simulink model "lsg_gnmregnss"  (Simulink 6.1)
settings: Solver=ode45  StartTime=0.0  StopTime=Tstop  MaxStep=step_max  RelTol=1e-3
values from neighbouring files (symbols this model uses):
  A = [ -RA/LA           -CE*PsiN/LA  ;         CM*PsiN/(2*pi*J) 0           ;      ]    [lsg_gnmregnss_ini.m]
  B = [  1/LA    0          ;         0      -1/(2*pi*J) ;      ]    [lsg_gnmregnss_ini.m]
  C = [  1  0 ;         0  1        ]    [lsg_gnmregnss_ini.m]
  CE = 2*pi*CM    (= 240.017678734)    [gnm_i.m]
  CM = 38.2    [gnm_i.m]
  D = zeros(size(C*B))    [lsg_gnmregnss_ini.m]
  int_regi = 0    [gnmregi_i.m]
  int_regn = 0    [lsg_gnmregnss_ini.m]    (also in gnmregn_i.m)
  J = 0.012    [gnm_i.m]
  MW = 0    [gnm_i.m]    (also in lsg_gnmregnss_ini.m = 100; gnmbeobreg_i.m = 10; gnmbeob_i.m = 10; gnmregn_i.m = 100)
  N_soll = 500/60    (= 8.33333333333)    [lsg_gnmregnss_ini.m]    (also in gnmbeobreg_i.m; gnmregn_i.m)
  PsiN = 0.04    [gnm_i.m]
  RA = 0.250    (= 0.25)    [gnm_i.m]
  T_MW = 0    [gnm_i.m]    (also in lsg_gnmregnss_ini.m = 0.1; gnmbeobreg_i.m = 0.4; gnmbeob_i.m = 0.4; gnmregn_i.m = 0.1)
  T_Nsoll = 0.40    (= 0.4)    [lsg_gnmregnss_ini.m]    (also in gnmbeobreg_i.m = 0.8; gnmregn_i.m)
  T_Ri = TA    [gnmregi_i.m]
  T_Rn = 4^2*2*T_t    [lsg_gnmregnss_ini.m]    (also in gnmregn_i.m = 4*2*T_t)
  T_t = 0.0001    [gnmregi_i.m]    (also in gnmbeobreg_i.m; gnmbeob_i.m)
  TA = LA / RA    (= 0.016)    [gnm_i.m]
  V_Ri = LA / (2*T_t)    [gnmregi_i.m]
  V_Rn = 2*pi*J / (CM*PsiN*4*2*T_t)    [lsg_gnmregnss_ini.m]    (also in gnmregn_i.m = 2*pi*J / (CM*PsiN*2*2*T_t))

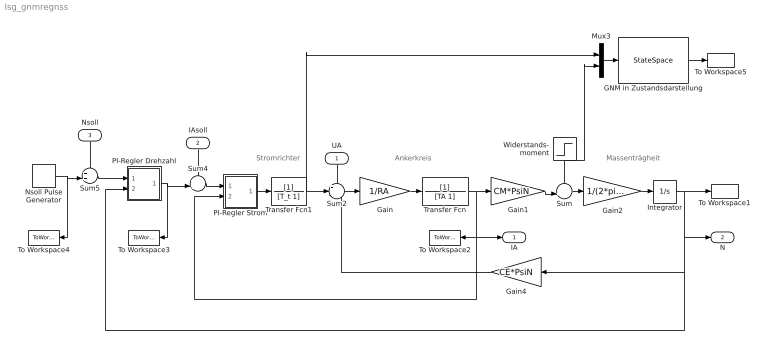
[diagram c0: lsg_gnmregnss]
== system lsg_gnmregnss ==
  note: Massenträgheit
  note: Ankerkreis
  note: Stromrichter
  UA : Inport  Orientation=down  Port=1  LatchInput=off
  IAsoll : Inport  Orientation=down  Port=2  PortDimensions=1  LatchInput=off
  Nsoll : Inport  Orientation=down  Port=3  PortDimensions=1  LatchInput=off
  GNM in Zustandsdarstellung : StateSpace  A=A  B=B  C=C  D=D
  Gain : Gain  Gain=1/RA
  Gain1 : Gain  Gain=CM*PsiN
  Gain2 : Gain  Gain=1/(2*pi*J)
  Gain4 : Gain  Orientation=left  Gain=CE*PsiN
  Integrator : Integrator
  Mux3 : Mux  Inputs=2
  Nsoll Pulse Generator : DiscretePulseGenerator  PulseType=Time based  Amplitude=N_soll  Period=T_Nsoll  PulseWidth=50
  PI-Regler Drehzahl : Subsystem  mask(PI-Regler){V_R=V_Rn, T_n=T_Rn, int_R=int_regn}
      mask prompts: V_R "Verstärkungsfaktor V_R"; T_n "Nachstellzeit T_n"; int_R "Startwert Regler-Integrator"
      mask help: 1 + s*T_n 1 + s*T_n Übertragungsfunktion: G_R = V_R * ------------------ = K_R * ------------------ s*T_n s
  PI-Regler Strom : Subsystem  mask(PI-Regler){V_R=V_Ri, T_n=T_Ri, int_R=int_regi}
      mask prompts: V_R "Verstärkungsfaktor V_R"; T_n "Nachstellzeit T_n"; int_R "Startwert Regler-Integrator"
      mask help: 1 + s*T_n 1 + s*T_n Übertragungsfunktion: G_R = V_R * ------------------ = K_R * ------------------ s*T_n s
  Sum : Sum  Inputs=-+|
  Sum2 : Sum  Inputs=++-
  Sum4 : Sum  Inputs=++|
  Sum5 : Sum  Inputs=++|
  To Workspace1 : ToWorkspace  VariableName=N  SampleTime=-1  SaveFormat=Array
  To Workspace2 : ToWorkspace  VariableName=IA  SampleTime=-1  SaveFormat=Array
  To Workspace3 : ToWorkspace  VariableName=IAsoll  SampleTime=-1  SaveFormat=Array
  To Workspace4 : ToWorkspace  VariableName=Nsoll  SampleTime=-1  SaveFormat=Array
  To Workspace5 : ToWorkspace  VariableName=yss  SampleTime=-1  SaveFormat=Array
  Transfer Fcn : TransferFcn  Denominator=[TA 1]
  Transfer Fcn1 : TransferFcn  Denominator=[T_t 1]
  Widerstands- moment : Step  Orientation=down  Time=T_MW  After=MW  SampleTime=0
  IA : Outport
  N : Outport  Port=2
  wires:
  PI-Regler Strom/1(Reglerausgang) -> Transfer Fcn1/1
  Gain/1 -> Transfer Fcn/1
  Sum2/1 -> Gain/1
  Gain1/1 -> Sum/2
  Widerstands- moment/1 -> Sum/1, Mux3/2
  Sum/1 -> Gain2/1
  Gain2/1 -> Integrator/1
  Integrator/1 -> To Workspace1/1, N/1, Gain4/1, PI-Regler Drehzahl/2(Istwert)
  UA/1 -> Sum2/1
  Gain4/1 -> Sum2/3
  Transfer Fcn/1 -> To Workspace2/1, IA/1, PI-Regler Strom/2(Istwert), Gain1/1
  Transfer Fcn1/1 -> Sum2/2, Mux3/1
  IAsoll/1 -> Sum4/1
  Sum4/1 -> PI-Regler Strom/1(Sollwert)
  PI-Regler Drehzahl/1(Reglerausgang) -> Sum4/2, To Workspace3/1
  Nsoll/1 -> Sum5/1
  Sum5/1 -> PI-Regler Drehzahl/1(Sollwert)
  Nsoll Pulse Generator/1 -> To Workspace4/1, Sum5/2
  GNM in Zustandsdarstellung/1 -> To Workspace5/1
  Mux3/1 -> GNM in Zustandsdarstellung/1

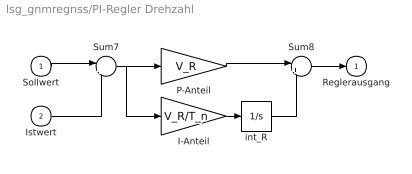
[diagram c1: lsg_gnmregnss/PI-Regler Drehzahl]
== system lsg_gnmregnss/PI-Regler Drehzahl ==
  Sollwert : Inport  Port=1  LatchInput=off
  Istwert : Inport  Port=2  LatchInput=off
  I-Anteil : Gain  Gain=V_R/T_n
  P-Anteil : Gain  Gain=V_R
  Sum7 : Sum  Inputs=|+-
  Sum8 : Sum  Inputs=|++
  int_R : Integrator  InitialCondition=int_R
  Reglerausgang : Outport  InitialOutput=0
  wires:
  P-Anteil/1 -> Sum8/1
  I-Anteil/1 -> int_R/1
  int_R/1 -> Sum8/2
  Sum8/1 -> Reglerausgang/1
  Sum7/1 -> P-Anteil/1, I-Anteil/1
  Istwert/1 -> Sum7/2
  Sollwert/1 -> Sum7/1

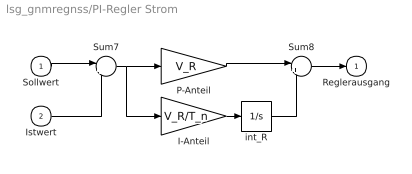
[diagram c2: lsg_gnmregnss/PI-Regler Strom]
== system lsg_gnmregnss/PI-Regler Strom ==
  Sollwert : Inport  Port=1  LatchInput=off
  Istwert : Inport  Port=2  LatchInput=off
  I-Anteil : Gain  Gain=V_R/T_n
  P-Anteil : Gain  Gain=V_R
  Sum7 : Sum  Inputs=|+-
  Sum8 : Sum  Inputs=|++
  int_R : Integrator  InitialCondition=int_R
  Reglerausgang : Outport  InitialOutput=0
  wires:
  P-Anteil/1 -> Sum8/1
  I-Anteil/1 -> int_R/1
  int_R/1 -> Sum8/2
  Sum8/1 -> Reglerausgang/1
  Sum7/1 -> P-Anteil/1, I-Anteil/1
  Istwert/1 -> Sum7/2
  Sollwert/1 -> Sum7/1
